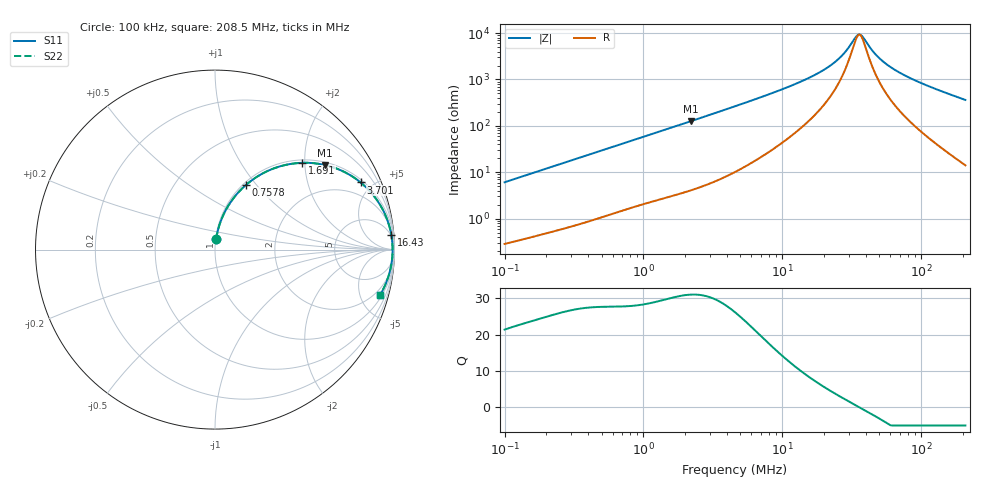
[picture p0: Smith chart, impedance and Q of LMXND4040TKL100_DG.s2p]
! LMXND4040TKL100_DG  S-PARAMETER MODEL  ( General Type )
! Model Generated by TAIYO YUDEN Corporation (http://www.ty-top.com)
! Version 1.0
! TAIYO YUDEN Control No. 191023NI43SB-FBB
! Copyright(c) 2019 TAIYO YUDEN CO.,LTD. All Rights Reserved.
! Product Description (link to TY-COMPAS)
! https://ds.yuden.co.jp/TYCOMPAS/or/detail?pn=LMXND4040TKL100MDG&u=M
! Products Name : Inductors
! Characteristics :
!  Inductance : 10 uH , SRF(min) : 25 MHz , DC Resistance(max) : 0.18 Ohm
!  Rated Current : Saturation :1300 mA , Temp Rise : 1200 mA
!  Case Size : 4.0 x 4.0 / 0.157 x 0.157 [mm/inch] , Thickness : 1.8 / 0.071 [mm/inch]
!  (Conditions: Temperature = 25 degC , DC Bias Current/Voltage = 0A / 0V)
! External Node Assignments :
!  1  o---GGG---o  2
! GND o---------o GND
! Frequency Range : 0.1MHz  -  208.503118MHz  [ 402 STEP ]
# MHz S RI R 50
! Freq[MHz].  S11 Real  S11 Imag  S21 Real  S21 Imag  S12 Real  S12 Imag  S22 Real  S22 Imag
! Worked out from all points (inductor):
!   401 points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, 100 kHz to 208.5 MHz, reference 50 ohm
!   read as one part in series: L = 9.64 uH near 103.9 kHz
!   highest Q = 31 at 2.209 MHz (marker M1), where L = 9.14 uH
!   self-resonance near 35.27 MHz
!   S11 on the Smith chart (normalised r, x): 100 kHz: 1.01, +0.12; 757.8 kHz: 1.03, +0.89; 1.691 MHz: 1.06, +1.95; 3.701 MHz: 1.15, +4.26; 16.43 MHz: 4, +23; 208.5 MHz: 1.28, -7.24
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0.1  0.0065 0.0603  0.9935 -0.0603  0.9935 -0.0603  0.0065 0.0603
0.198939  0.0186 0.1166  0.9814 -0.1166  0.9814 -0.1166  0.0186 0.1166
0.359709  0.0504 0.2011  0.9496 -0.2011  0.9496 -0.2011  0.0504 0.2011
0.757818  0.1727 0.3604  0.8273 -0.3604  0.8273 -0.3604  0.1727 0.3604
1.293906  0.3632 0.4641  0.6368 -0.4641  0.6368 -0.4641  0.3632 0.4641
1.69072  0.4869 0.4836  0.5131 -0.4836  0.5131 -0.4836  0.4869 0.4836
2.209228  0.6135 0.4711  0.3865 -0.4711  0.3865 -0.4711  0.6135 0.4711
3.700673  0.8114 0.3742  0.1886 -0.3742  0.1886 -0.3742  0.8114 0.3742
4.654297  0.8697 0.3178  0.1303 -0.3178  0.1303 -0.3178  0.8697 0.3178
9.619882  0.9616 0.1612  0.0384 -0.1612  0.0384 -0.1612  0.9616 0.1612
16.42508  0.9823 0.0822  0.0177 -0.0822  0.0177 -0.0822  0.9823 0.0822
20.65765  0.9862 0.0555  0.0138 -0.0555  0.0138 -0.0555  0.9862 0.0555
25.00684  0.9881 0.0354  0.0119 -0.0354  0.0119 -0.0354  0.9881 0.0354
28.58534  0.9889 0.022  0.0111 -0.022  0.0111 -0.022  0.9889 0.022
33.94871  0.9894 0.00537  0.0106 -0.00537  0.0106 -0.00537  0.9894 0.00537
35.95147  0.9894 -0.000123  0.0106 0.000123  0.0106 0.000123  0.9894 -0.000123
38.07238  0.9894 -0.00562  0.0106 0.00562  0.0106 0.00562  0.9894 -0.00562
47.88322  0.9886 -0.028  0.0114 0.028  0.0114 0.028  0.9886 -0.028
59.08252  0.987 -0.0496  0.013 0.0496  0.013 0.0496  0.987 -0.0496
72.90118  0.984 -0.0733  0.016 0.0733  0.016 0.0733  0.984 -0.0733
97.09599  0.977 -0.1105  0.023 0.1105  0.023 0.1105  0.977 -0.1105
208.5031  0.9208 -0.2513  0.0792 0.2513  0.0792 0.2513  0.9208 -0.2513
